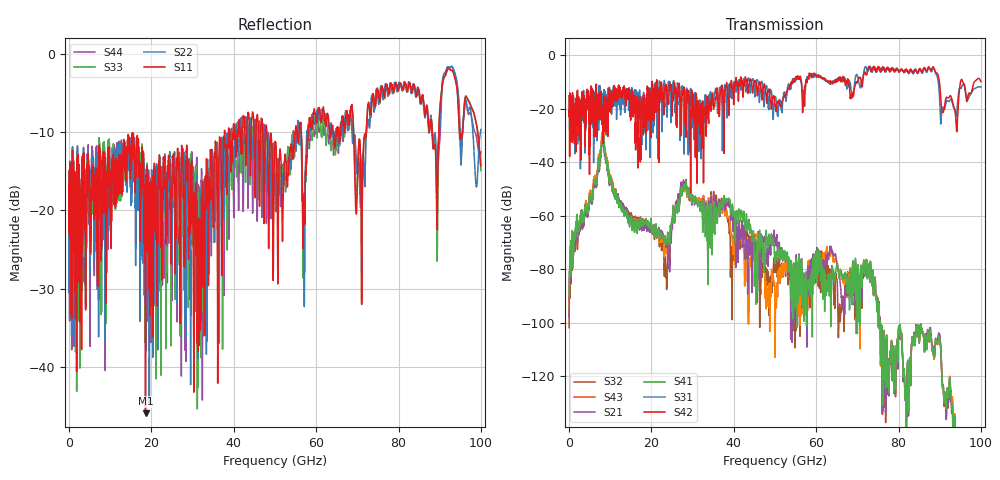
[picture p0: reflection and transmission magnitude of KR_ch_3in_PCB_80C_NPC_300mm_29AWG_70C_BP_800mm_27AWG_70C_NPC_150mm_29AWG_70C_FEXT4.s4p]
# Hz S RI R 45
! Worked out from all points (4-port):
!   4000 points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, 25 MHz to 100 GHz, reference 45 ohm
!   strongest paths, dB at 25 MHz, 25.02 GHz, 50.02 GHz, 75.03 GHz, 100 GHz:
!     S42: -20.7, -20.7, -18.8, -4.2, -9.7
!     S31: -20.6, -14.0, -16.0, -5.1, -11.8
!     S41: -90.5, -61.8, -77.0, -99.7, -178.7
!     S21: -97.9, -64.2, -69.4, -99.0, -175.2
!     S43: -97.2, -61.9, -96.1, -99.6, -177.5
!     S32: -101.9, -62.0, -79.4, -98.8, -174.6
!   lowest |S11| = -45.9 dB at 18.57 GHz (marker M1), VSWR 1.01, Z = 45.4 + j0.0957 ohm
!   |S11| at or under -10 dB: start of sweep to 37.74 GHz; 48.05 GHz to 54.87 GHz (6.818 GHz wide, 13.2 % of centre); 69.09 GHz to 72.19 GHz (3.1 GHz wide, 4.39 % of centre)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
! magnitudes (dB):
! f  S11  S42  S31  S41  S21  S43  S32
! 25 MHz  -16.6  -20.7  -20.6  -90.5  -97.9  -97.2  -101.9
! 8.15 GHz  -19.2  -21.4  -18.8  -30.5  -32.3  -28.5  -30.1
! 18.57 GHz  -45.9  -20.1  -21.0  -61.7  -63.8  -62.1  -62.4
! 23.5 GHz  -18.2  -12.4  -14.0  -70.0  -71.5  -72.9  -80.5
! 28 GHz  -25.4  -13.4  -25.0  -49.5  -48.4  -50.4  -49.4
! 45.95 GHz  -9.3  -11.7  -10.5  -67.4  -80.3  -66.1  -73.5
! 100 GHz  -14.3  -9.7  -11.8  -178.7  -175.2  -177.5  -174.6
